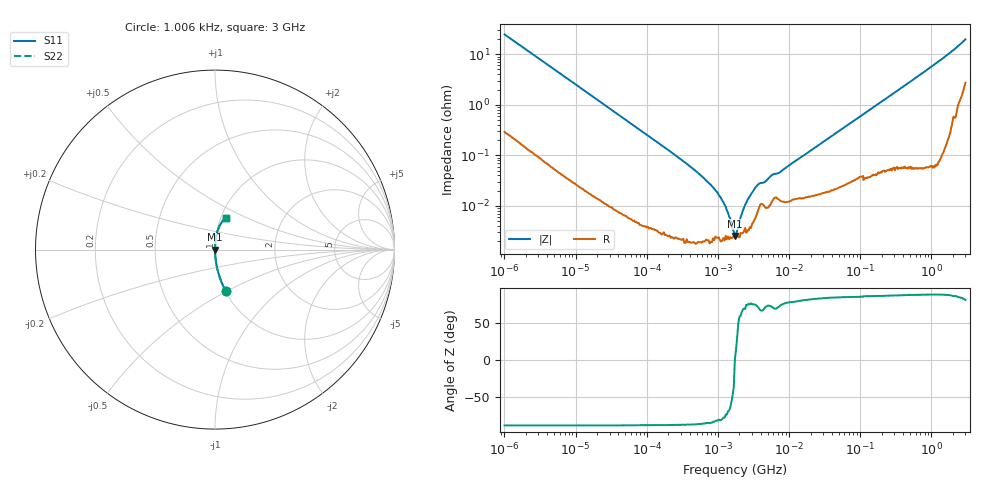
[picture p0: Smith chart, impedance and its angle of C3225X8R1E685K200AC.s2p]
! S-Parameter Data Generated by TDK Corporation
! Copyright(C) 2022 TDK Corporation.
! All Rights Reserved.
! TDK P/N: C3225X8R1E685K200AC (Multilayer Ceramic Chip Capacitor)
! Property: C=6.8uF
! Size(LxWxT): 3.2x2.5x2mm
! Model Type: s2p (Touchstone File Format Version 1.0)
! Frequency: DC=Yes Start=0.00100604MHz Stop=3000MHz 481points Log-sweep
! Model Generated on Apr. 15, 2022
! Port Assignments:
!  1 ---| |--- 2
! Applicable Conditions:
!  Temperature = 25 degC
!  DC Bias Voltage = 0 V
!  Small Signal Operation
! Terms and conditions regarding TDK Simulation Models
! (1)This simulation model is being provided solely for informational purposes. Please refer to the specifications of the products in terms of detailed characteristics of such products.
! (2)In no event shall TDK Corporation of any of its subsidiaries be liable for any loss or damage arising, directly or indirectly,
!  From any information contained in this simulation model, including, but not limited to loss or damages arising from any inaccuracies, omissions or errors in connection with such information.
! (3)Any and all copyrights on this simulation model are owned by TDK Corporation.
!  Duplication or redistribution of this simulation model without prior written permission from TDK Corporation is prohibited.
! (4)This simulation model is subject to any modification or change without any prior notice.
! (5)Neither TDK Corporation nor any of its subsidiaries shall make any warranty, express or implied,
!  Including but not limited to the correctness, implied warranties of merchantability and fitness for a particular purpose with respect to this simulation models.
! (6)The use of this simulation model shall be deemed to have consented to the terms and conditions hereof.
# Hz S MA R 50
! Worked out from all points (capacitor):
!   480 points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, 1.006 kHz to 3 GHz, reference 50 ohm
!   read as one part in series: C = 6.41 uF near 1.083 kHz
!   lowest |Z| = 2.54 mohm at 1.731 MHz (marker M1)
!   series resonance near 1.73 MHz, so ESL is about 1.3 nH
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1006.04  0.2382 -75.5  0.9684 13.8  0.9684 13.8  0.2382 -75.5
2947.59  0.0846 -84.5  0.9955 4.9  0.9955 4.9  0.0846 -84.5
12511.3  0.02026 -88.2  0.9996 1.2  0.9996 1.2  0.02026 -88.2
149930  0.001707 -88.9  1 0.1  1 0.1  0.001707 -88.9
351683  0.0007059 -88.4  1 0.0  1 0.0  0.0007059 -88.4
590919  0.0003872 -87.2  1 0.0  1 0.0  0.0003872 -87.2
921951  0.0002023 -83.0  1 0.0  1 0.0  0.0002023 -83.0
1287040  9.56e-05 -74.5  1 0.0  1 0.0  9.56e-05 -74.5
1731330  2.538e-05 0.9  1 -0.0  1 -0.0  2.538e-05 0.9
1796710  2.721e-05 14.4  1 -0.0  1 -0.0  2.721e-05 14.4
2328980  9.319e-05 70.2  1 -0.0  1 -0.0  9.319e-05 70.2
2508200  0.0001161 75.3  1 -0.0  1 -0.0  0.0001161 75.3
3132950  0.0001987 76.2  1 -0.0  1 -0.0  0.0001987 76.2
3633680  0.0002617 72.6  0.9999 -0.0  0.9999 -0.0  0.0002617 72.6
4538750  0.0002968 71.0  0.9999 -0.0  0.9999 -0.0  0.0002968 71.0
5883350  0.0004157 72.0  0.9999 -0.0  0.9999 -0.0  0.0004157 72.0
7626280  0.0004751 74.9  0.9999 -0.0  0.9999 -0.0  0.0004751 74.9
2.15311e7  0.001326 83.1  0.9998 -0.1  0.9998 -0.1  0.001326 83.1
2.50734e8  0.01443 87.1  0.9994 -0.8  0.9994 -0.8  0.01443 87.1
1.1478e9  0.06509 85.7  0.9972 -3.7  0.9972 -3.7  0.06509 85.7
2.17789e9  0.1289 80.1  0.9861 -7.4  0.9861 -7.4  0.1289 80.1
3e9  0.1884 71.3  0.9563 -10.8  0.9563 -10.8  0.1884 71.3
